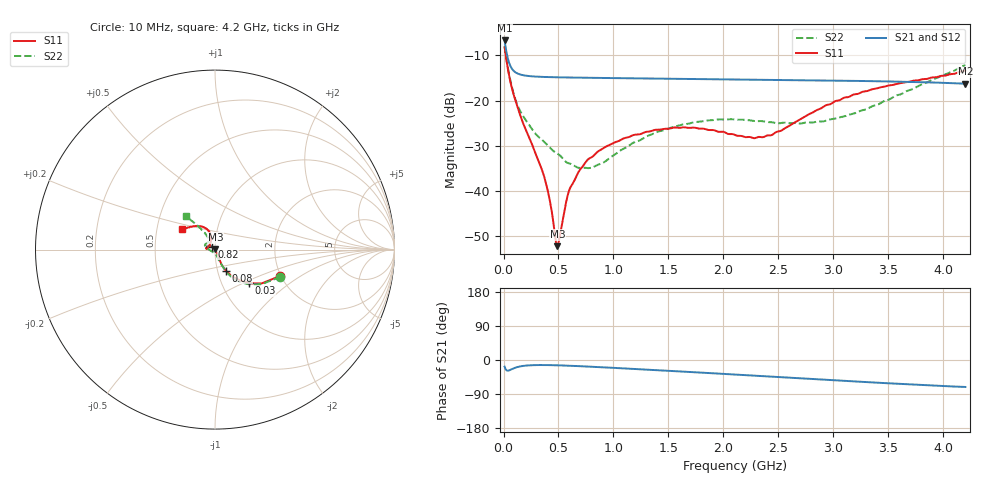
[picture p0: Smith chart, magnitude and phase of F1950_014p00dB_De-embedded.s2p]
! Integrated Device Technology
! Corporate Headquarters
! 6024 Silver Creek Valley Road
! San Jose, CA 95138  USA
! Phone:  1-408-284-8200
! Toll Free:  1-800-223-1366
! Webpage:  http://www.idt.com/
! Timing and RF Division
! 515 Groton Road, Suite 102
! Westford, MA 01886-6024
! Device:  F1950
! Description: 7-bit 0.25 dB Digital Step Attenuator
! Frequency:  150.0 -  4000.00 MHz
! Package:  4x4 mm Thin QFN Plastic Package: 24 pin
! Ports:  2 RF, 12 DC
!  Pin  1  = D0
!  Pin  2  = VDD
!  Pin  3  = Vmode
!  Pin  4  = GND
!  Pin  5  = RF1  =  Port 1
!  Pin  6  = GND
!  Pin  7  = GND
!  Pin  8  = GND
!  Pin  9  = GND
!  Pin 10  = GND
!  Pin 11  = GND
!  Pin 12  = GND
!  Pin 13  = GND
!  Pin 14  = RF2  =  Port 2
!  Pin 15  = GND
!  Pin 16  = LE
!  Pin 17  = CLK
!  Pin 18  = DATE
!  Pin 19  = D6
!  Pin 20  = D5
!  Pin 21  = D4
!  Pin 22  = D3
!  Pin 23  = D2
!  Pin 24  = D1
! State:  56
! Atten State:  14.00 dB
! Voltage:  +5.00 Volts
! Current:  Not Measured mA
! Data:  The device was measured on a the F195X evaluation board which has
!  individual transmission lines to the RF pins.  Data was collected
!  using a calibrated network analyzer.  The evaluation board was
!  de-embedded using a TRL calibration technique.
!  The reference plane is the edge of the package pin.
! Misc:  Board 2019
!  Action Tracker AT0250
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# GHz S dB R 50
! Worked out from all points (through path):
!   420 points, 10 MHz to 4.2 GHz, reference 50 ohm
!   highest |S21| = -6.69 dB at 10 MHz (marker M1); lowest = -16.3 dB at 4.2 GHz (marker M2)
!   group delay of S21, straight-line fit = 41.3 ps
!   lowest |S11| = -52.2 dB at 490 MHz (marker M3), VSWR 1.00, Z = 50.2 + j0.174 ohm
!   |S11| at or under -10 dB: 20.69 MHz to end of sweep
!   |S22| runs from -34.9 to -8.1 dB; largest |S21 - S12| = 0.00025
!   S11 on the Smith chart (normalised r, x): 10 MHz: 1.98, -0.69; 30 MHz: 1.34, -0.54; 80 MHz: 1.10, -0.26; 820 MHz: 0.96, +0.03; 4.2 GHz: 0.68, +0.16
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0.01  -8.16 -22.1  -6.69 -17.5  -6.69 -17.5  -8.09 -22.7
0.03  -11.52 -44.7  -9.64 -27.7  -9.64 -27.7  -11.39 -45.8
0.05  -14.36 -55.2  -11.57 -27.5  -11.57 -27.5  -14.10 -56.4
0.08  -17.60 -62.8  -13.07 -23.5  -13.07 -23.5  -17.37 -63.1
0.17  -24.47 -65.2  -14.33 -16.0  -14.33 -16.0  -23.10 -69.7
0.37  -36.80 -49.4  -14.77 -13.3  -14.76 -13.3  -29.11 -75.5
0.42  -41.93 -42.1  -14.80 -13.5  -14.80 -13.5  -30.34 -77.3
0.47  -50.05 -1.7  -14.83 -13.8  -14.83 -13.8  -31.43 -83.3
0.49  -52.18 44.8  -14.84 -14.0  -14.84 -14.0  -31.72 -85.1
0.51  -50.21 83.2  -14.85 -14.2  -14.85 -14.2  -32.06 -86.2
0.59  -40.37 119.5  -14.88 -15.0  -14.88 -15.0  -33.82 -97.2
0.71  -34.85 131.6  -14.92 -16.5  -14.92 -16.5  -34.86 -117.4
0.82  -32.18 138.1  -14.96 -18.1  -14.96 -18.1  -34.65 -139.4
1.09  -28.37 153.3  -15.04 -22.0  -15.04 -22.1  -30.66 -173.9
1.41  -26.42 166.9  -15.13 -27.1  -15.13 -27.1  -26.83 170.6
1.73  -25.96 173.8  -15.21 -32.2  -15.20 -32.2  -24.79 161.5
2.11  -27.64 164.8  -15.30 -38.5  -15.30 -38.5  -24.20 152.4
2.43  -27.67 131.2  -15.39 -43.7  -15.39 -43.7  -24.76 142.9
2.81  -22.65 107.3  -15.49 -50.1  -15.49 -50.2  -24.83 128.2
3.19  -18.61 110.5  -15.62 -56.5  -15.62 -56.6  -22.83 121.0
3.51  -16.62 119.5  -15.76 -61.6  -15.76 -61.7  -19.71 121.4
4.2  -13.34 147.7  -16.25 -71.2  -16.25 -71.2  -12.12 130.9
